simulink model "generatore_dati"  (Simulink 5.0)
settings: Solver=ode45  StartTime=0.0  StopTime=1000  RelTol=1e-3
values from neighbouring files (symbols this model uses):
  Kd = 1    [test.m]
  Kstoc = 1    [test.m]
  Ku = 1    [test.m]
  pd = [.5]    [test.m]
  ps = [-.9 .9]    [test.m]
  pu = [.9]    [test.m]
  seed1 = 10000*rand    [test.m]
  seed2 = randn    [test.m]
  zd = []    [test.m]
  zs = [-j*.99 j*.99]    [test.m]
  zu = [-.9]    [test.m]

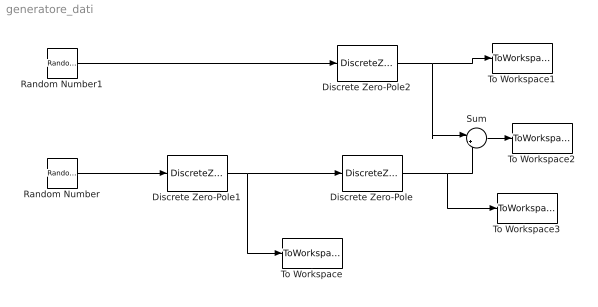
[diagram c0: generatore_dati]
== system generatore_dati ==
  Discrete Zero-Pole : DiscreteZeroPole  Zeros=[zd]  Poles=[pd]  Gain=Kd
  Discrete Zero-Pole1 : DiscreteZeroPole  Zeros=[zu]  Poles=[pu]  Gain=Ku
  Discrete Zero-Pole2 : DiscreteZeroPole  Zeros=[zs]  Poles=[ps]  Gain=Kstoc
  Random Number : RandomNumber  Seed=seed2  SampleTime=1
  Random Number1 : RandomNumber  Seed=seed1  SampleTime=1
  Sum : Sum  Inputs=|++
  To Workspace : ToWorkspace  VariableName=u  SampleTime=-1  SaveFormat=Array
  To Workspace1 : ToWorkspace  VariableName=ys  SampleTime=-1  SaveFormat=Array
  To Workspace2 : ToWorkspace  VariableName=y  SampleTime=-1  SaveFormat=Array
  To Workspace3 : ToWorkspace  VariableName=yd  SampleTime=-1  SaveFormat=Array
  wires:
  Random Number/1 -> Discrete Zero-Pole1/1
  Discrete Zero-Pole1/1 -> Discrete Zero-Pole/1, To Workspace/1
  Discrete Zero-Pole/1 -> Sum/2, To Workspace3/1
  Discrete Zero-Pole2/1 -> Sum/1, To Workspace1/1
  Sum/1 -> To Workspace2/1
  Random Number1/1 -> Discrete Zero-Pole2/1
